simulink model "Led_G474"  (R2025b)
settings: Solver=FixedStepAuto  StartTime=0.0  StopTime=10.0  RelTol=1e-3  EnableMultiTasking=on
libraries: stm32f4xxblockslib x3

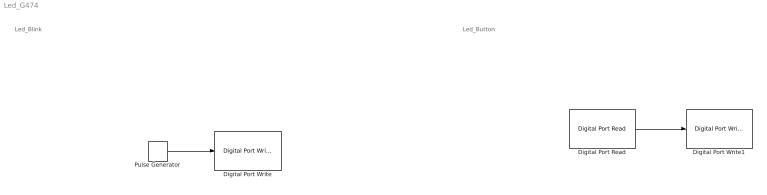
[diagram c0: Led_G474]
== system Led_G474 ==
  note: Led_Blink
  note: Led_Button
  Digital Port Read : stm32f4xxblockslib/Digital Port Read  PortName=GPIOC  PinNumber=[13]  ReadOperation=on  IOAsArray=on  SampleTime=-1  EnableSimPort=off  hoistedMaskSrc=ECSoC/ECSimCodegen/Digital Port Read
  Digital Port Write : stm32f4xxblockslib/Digital Port Write  Commented=on  PortName=GPIOA  PinNumber=[5]  ReadOperation=off  IOAsArray=on  EnableSimPort=off  hoistedMaskSrc=ECSoC/ECSimCodegen/Digital Port Write
  Digital Port Write1 : stm32f4xxblockslib/Digital Port Write  PortName=GPIOA  PinNumber=[5]  ReadOperation=off  IOAsArray=on  EnableSimPort=off  hoistedMaskSrc=ECSoC/ECSimCodegen/Digital Port Write
  Pulse Generator : DiscretePulseGenerator  Commented=on  PulseType=Time based  PulseWidth=50
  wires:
  Pulse Generator/1 -> Digital Port Write/1
  Digital Port Read/1 -> Digital Port Write1/1
